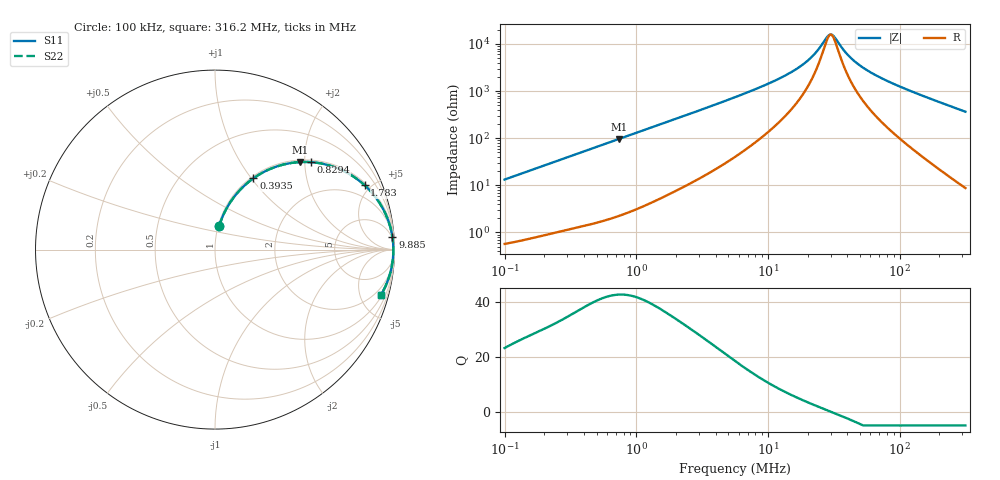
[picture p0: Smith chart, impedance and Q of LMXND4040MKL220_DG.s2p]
! LMXND4040MKL220_DG  S-PARAMETER MODEL  ( General Type )
! Model Generated by TAIYO YUDEN Corporation (https://www.yuden.co.jp/en/)
! Version 1.0
! TAIYO YUDEN Control No. 191023NI43SB-FBB
! Copyright(c) 2019 TAIYO YUDEN CO.,LTD. All Rights Reserved.
! Product Description (link to TY-COMPAS)
! https://ds.yuden.co.jp/TYCOMPAS/or/detail?pn=LMXND4040MKL220MDG&u=M
! Products Name : Inductors
! Characteristics :
!  Inductance : 22 uH , SRF(min) : 18 MHz , DC Resistance(max) : 0.48 Ohm
!  Rated Current : Saturation :500 mA , Temp Rise : 620 mA (40 degC)
!  Case Size : 4.0 x 4.0 / 0.157 x 0.157 [mm/inch] , Thickness : 1.2 / 0.047 [mm/inch]
!  (Conditions: Temperature = 25 degC , DC Bias Current/Voltage = 0A / 0V)
! External Node Assignments :
!  1  o---GGG---o  2
! GND o---------o GND
! Frequency Range : 0.1MHz  -  316.199832MHz  [ 402 STEP ]
# MHz S RI R 50
! Freq[MHz].  S11 Real  S11 Imag  S21 Real  S21 Imag  S12 Real  S12 Imag  S22 Real  S22 Imag
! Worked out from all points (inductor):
!   401 points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, 100 kHz to 316.2 MHz, reference 50 ohm
!   read as one part in series: L = 21 uH near 104.1 kHz
!   highest Q = 42.7 at 734.9 kHz (marker M1), where L = 20.6 uH
!   self-resonance near 29.94 MHz
!   S11 on the Smith chart (normalised r, x): 100 kHz: 1.01, +0.26; 393.5 kHz: 1.03, +1.02; 829.4 kHz: 1.05, +2.15; 1.783 MHz: 1.13, +4.60; 9.885 MHz: 4, +28; 316.2 MHz: 1.17, -7.30
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0.1  0.0226 0.1288  0.9774 -0.1288  0.9774 -0.1288  0.0226 0.1288
0.215029  0.0809 0.257  0.9191 -0.257  0.9191 -0.257  0.0809 0.257
0.385695  0.2077 0.3926  0.7923 -0.3926  0.7923 -0.3926  0.2077 0.3926
0.393544  0.214 0.3972  0.786 -0.3972  0.786 -0.3972  0.214 0.3972
0.734921  0.4758 0.4878  0.5242 -0.4878  0.5242 -0.4878  0.4758 0.4878
0.829354  0.5344 0.4872  0.4656 -0.4872  0.4656 -0.4872  0.5344 0.4872
1.487603  0.7803 0.401  0.2197 -0.401  0.2197 -0.401  0.7803 0.401
1.783349  0.834 0.3582  0.166 -0.3582  0.166 -0.3582  0.834 0.3582
2.9511  0.9281 0.2412  0.0719 -0.2412  0.0719 -0.2412  0.9281 0.2412
5.623165  0.9753 0.1304  0.0247 -0.1304  0.0247 -0.1304  0.9753 0.1304
9.885033  0.9885 0.0696  0.0115 -0.0696  0.0115 -0.0696  0.9885 0.0696
15.7118  0.9924 0.0358  0.00764 -0.0358  0.00764 -0.0358  0.9924 0.0358
21.68824  0.9934 0.0171  0.00658 -0.0171  0.00658 -0.0171  0.9934 0.0171
28.18209  0.9937 0.00326  0.00626 -0.00326  0.00626 -0.00326  0.9937 0.00326
30.54729  0.9938 -0.000914  0.00625 0.000914  0.00625 0.000914  0.9938 -0.000914
32.45058  0.9937 -0.00405  0.00626 0.00405  0.00626 0.00405  0.9937 -0.00405
39.69369  0.9936 -0.0147  0.00645 0.0147  0.00645 0.0147  0.9936 -0.0147
46.63594  0.9932 -0.0235  0.00679 0.0235  0.00679 0.0235  0.9932 -0.0235
59.39086  0.9923 -0.0381  0.00769 0.0381  0.00769 0.0381  0.9923 -0.0381
83.65039  0.9898 -0.0626  0.0102 0.0626  0.0102 0.0626  0.9898 -0.0626
153.0964  0.9778 -0.1249  0.0222 0.1249  0.0222 0.1249  0.9778 -0.1249
316.1998  0.9251 -0.2515  0.0749 0.2515  0.0749 0.2515  0.9251 -0.2515
